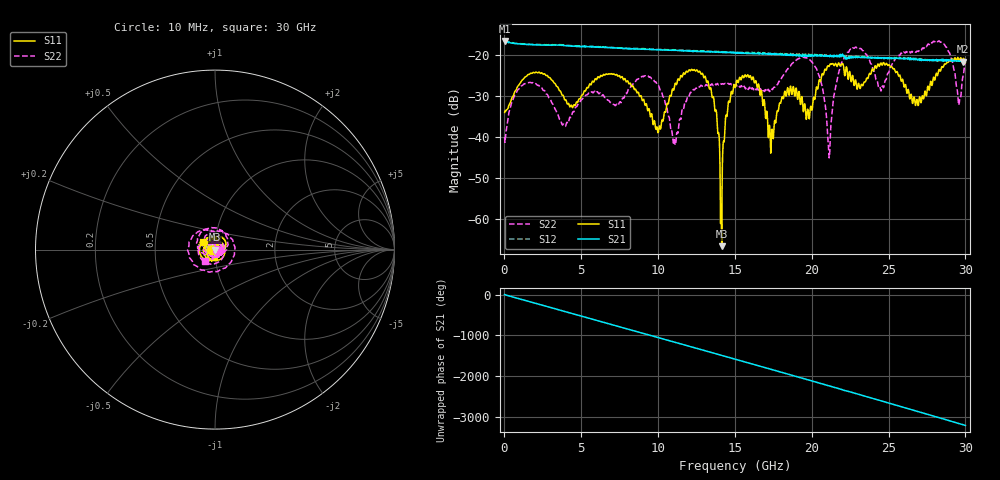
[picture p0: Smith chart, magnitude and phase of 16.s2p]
!Agilent Technologies,E8364B,US42250130,A.04.87.01
!Agilent E8364B: A.04.87.01
!Date: Monday, February 07, 2022 23:46:25
!Correction: S11(Full 2 Port SOLT,1,2) S21(Full 2 Port SOLT,1,2) S12(Full 2 Port SOLT,1,2) S22(Full 2 Port SOLT,1,2)
!S2P File: Measurements: S11, S21, S12, S22:
# Hz S  dB  R 50
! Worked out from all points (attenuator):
!   1601 points, 10 MHz to 30 GHz, reference 50 ohm
!   highest |S21| = -16.45 dB at 28.74 MHz (marker M1); lowest = -21.6 dB at 29.85 GHz (marker M2)
!   lowest |S11| = -66.7 dB at 14.14 GHz (marker M3), VSWR 1.00, Z = 50 + j0.0273 ohm
!   |S11| at or under -10 dB: start of sweep to end of sweep
!   |S22| runs from -45.1 to -16.3 dB; largest |S21 - S12| = 0.012
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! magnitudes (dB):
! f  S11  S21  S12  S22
! 10 MHz  -34.0  -16.6  -16.6  -40.0
! 28.74 MHz  -33.6  -16.5  -16.4  -41.3
! 1.36 GHz  -25.3  -17.3  -17.2  -26.9
! 3.852 GHz  -30.1  -17.6  -17.4  -36.8
! 5.015 GHz  -29.8  -17.9  -17.7  -30.8
! 7.376 GHz  -25.1  -18.2  -18.1  -32.2
! 10.02 GHz  -38.7  -18.6  -18.5  -27.4
! 11.07 GHz  -27.6  -18.8  -18.7  -40.6
! 12.77 GHz  -24.5  -19.1  -18.9  -27.4
! 13.67 GHz  -32.6  -19.1  -19.1  -26.9
! 14.14 GHz  -66.7  -19.1  -19.1  -27.1
! 15.01 GHz  -27.7  -19.3  -19.2  -27.3
! 16.28 GHz  -26.7  -19.5  -19.3  -28.0
! 17.33 GHz  -43.9  -19.6  -19.5  -28.2
! 18.51 GHz  -29.7  -20.0  -19.6  -22.9
! 20.01 GHz  -33.4  -19.9  -19.9  -21.6
! 21.12 GHz  -22.7  -20.1  -20.2  -43.8
! 22.41 GHz  -25.1  -20.5  -20.2  -19.2
! 25.01 GHz  -22.3  -20.8  -20.7  -24.2
! 26.85 GHz  -30.8  -21.0  -20.9  -18.9
! 29.85 GHz  -20.9  -21.6  -21.0  -25.0
! 30 GHz  -21.7  -21.4  -21.2  -21.2
